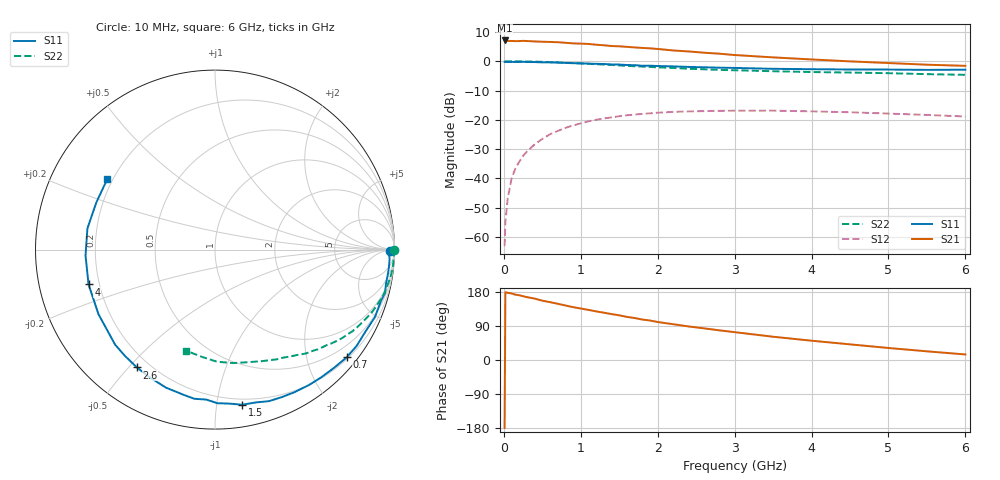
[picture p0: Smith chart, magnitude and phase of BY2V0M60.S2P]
! SIEMENS Small Signal Semiconductors
! BFY420
! Si NPN RF SIEGET Grounded Emitter Transistor in MICRO-X
! VCE = 2 V  IC = 0.6 mA
! Common Emitter S-Parameters:  October  1996
# GHz  S  MA  R  50
!  f  S11  S21  S12  S22
! GHz  MAG  ANG  MAG  ANG  MAG  ANG  MAG  ANG
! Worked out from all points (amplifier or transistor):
!   36 points, 10 MHz to 6 GHz, reference 50 ohm
!   highest |S21| = 7.1 dB at 10 MHz (marker M1)
!   |S21| within 3 dB of that: start of sweep to 2.038 GHz
!   unconditionally stable (mu >= 1): 4.721 GHz to end of sweep
!   at 250 MHz: K = 0.03, MSG = 19.6 dB, |S12| = -32.3 dB
!   at 1.4 GHz: K = 0.18, MSG = 12.2 dB, |S12| = -19.2 dB
!   at 6 GHz: K = 1.40, MAG = 4.9 dB, |S12| = -18.9 dB
!   S11 on the Smith chart (normalised r, x): 10 MHz: 69, -30; 700 MHz: 0.24, -2.78; 1.5 GHz: 0.16, -1.18; 2.6 GHz: 0.15, -0.53; 4 GHz: 0.16, -0.13; 6 GHz: 0.18, +0.29
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0.01  0.976 -0.6  2.26 -179.2  0.0007 96.8  0.9999 -0.2
0.02  0.9688 -1.3  2.241 178.9  0.0018 92.4  0.9936 -0.5
0.05  0.9744 -3.1  2.209 177.2  0.0045 85.8  0.9988 -1.4
0.1  0.974 -5.9  2.219 175.8  0.0099 87.9  0.9948 -2.8
0.15  0.9727 -8.6  2.202 172.4  0.0148 83.3  0.9958 -4.2
0.25  0.9778 -14.3  2.224 168.3  0.0243 80.4  0.9931 -6.9
0.4  0.9673 -22.9  2.175 162.1  0.038 75.9  0.9831 -11.0
0.5  0.9548 -28.4  2.149 156.5  0.0473 72.7  0.9759 -13.7
0.7  0.9478 -39.3  2.11 148.4  0.0645 65.5  0.9543 -18.9
0.9  0.9259 -50.0  2.016 139.5  0.0803 58.2  0.9291 -23.8
1.1  0.9096 -60.8  1.971 132.2  0.0942 52.0  0.9033 -28.5
1.5  0.8776 -80.0  1.796 117.9  0.1151 40.2  0.8486 -36.8
1.8  0.837 -93.3  1.686 106.8  0.1262 32.7  0.8097 -42.1
1.9  0.839 -97.9  1.657 104.1  0.1293 30.3  0.7984 -44.1
2.2  0.816 -109.6  1.526 94.5  0.1366 23.6  0.7685 -48.9
2.6  0.7877 -123.5  1.398 83.6  0.1409 16.1  0.7286 -54.8
3  0.7683 -136.4  1.275 73.5  0.1431 9.7  0.7015 -60.6
3.5  0.7423 -151.0  1.163 61.4  0.1434 2.8  0.6749 -67.0
4  0.7307 -164.6  1.072 50.9  0.1396 -2.8  0.6534 -73.8
4.5  0.7221 -177.3  0.994 41.3  0.1347 -7.6  0.6402 -80.9
5.5  0.7114 158.3  0.872 22.9  0.1213 -12.8  0.6019 -97.0
6  0.7171 146.9  0.834 14.6  0.1139 -13.0  0.5859 -106.0
